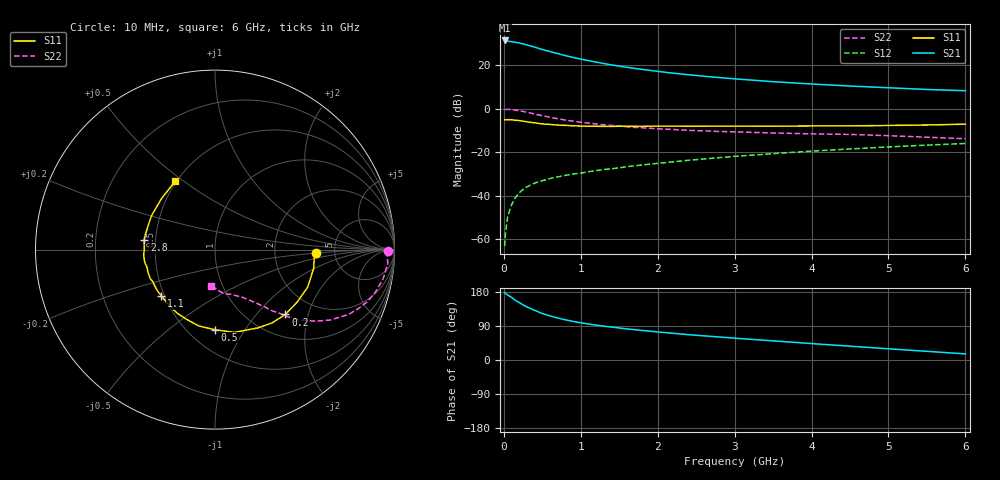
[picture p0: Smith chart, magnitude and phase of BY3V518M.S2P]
! SIEMENS Small Signal Semiconductors
! BFY420
! Si NPN RF SIEGET Grounded Emitter Transistor in MICRO-X
! VCE = 3.5 V  IC = 18 mA
! Common Emitter S-Parameters:  October  1996
# GHz  S  MA  R  50
!  f  S11  S21  S12  S22
! GHz  MAG  ANG  MAG  ANG  MAG  ANG  MAG  ANG
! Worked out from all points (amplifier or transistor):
!   36 points, 10 MHz to 6 GHz, reference 50 ohm
!   highest |S21| = 31.3 dB at 10 MHz (marker M1)
!   |S21| within 3 dB of that: start of sweep to 395.2 MHz
!   unconditionally stable (mu >= 1): start of sweep to 12.51 MHz; 2.07 GHz to end of sweep
!   at 250 MHz: K = 0.29, MSG = 33.4 dB, |S12| = -37.1 dB
!   at 1.4 GHz: K = 0.89, MSG = 23.8 dB, |S12| = -27.6 dB
!   at 6 GHz: K = 1.06, MAG = 10.6 dB, |S12| = -16.0 dB
!   S11 on the Smith chart (normalised r, x): 10 MHz: 3.55, -0.21; 200 MHz: 1.43, -1.45; 500 MHz: 0.67, -0.74; 1.1 GHz: 0.48, -0.29; 2.8 GHz: 0.43, +0.06; 6 GHz: 0.49, +0.46
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0.01  0.5616 -2.1  36.71 178.4  0.0007 72.9  0.9626 -0.5
0.02  0.5546 -4.5  36.18 175.7  0.0013 71.8  0.9589 -1.4
0.1  0.5572 -22.1  34.53 165.2  0.0062 80.8  0.951 -9.8
0.15  0.543 -32.6  33.32 157.4  0.0091 71.7  0.9268 -14.5
0.2  0.5334 -42.6  32.09 151.7  0.0118 72.0  0.8983 -18.7
0.25  0.5174 -52.2  30.55 145.3  0.014 69.2  0.8616 -22.6
0.3  0.4976 -61.2  28.98 139.9  0.0161 67.3  0.8267 -25.9
0.4  0.4736 -76.8  25.85 131.1  0.0196 63.4  0.7528 -31.4
0.5  0.4461 -90.2  22.76 122.6  0.0222 60.1  0.6883 -35.4
0.6  0.435 -101.9  20.4 116.4  0.0249 58.4  0.634 -38.5
0.7  0.4206 -111.2  18.36 110.8  0.0272 58.6  0.5882 -41.1
0.8  0.413 -119.9  16.49 106.0  0.0294 56.8  0.5479 -42.9
0.9  0.4056 -126.6  14.96 101.9  0.0317 56.9  0.5159 -44.1
1.1  0.395 -139.2  12.67 95.0  0.0357 57.0  0.4661 -47.0
1.3  0.3924 -148.3  10.84 89.3  0.0402 57.0  0.4275 -48.7
1.6  0.3943 -160.2  8.885 82.0  0.0466 57.4  0.3838 -51.7
2.2  0.3987 -175.9  6.518 70.5  0.0602 56.5  0.3329 -56.7
2.8  0.3982 172.1  5.172 60.7  0.0752 54.1  0.2989 -61.3
3.5  0.3959 159.7  4.159 50.5  0.0928 50.2  0.2767 -66.7
4.5  0.4026 144.4  3.301 36.5  0.1189 42.8  0.2561 -75.2
5.5  0.4223 127.9  2.754 22.9  0.1457 34.3  0.2214 -87.7
6  0.4405 120.4  2.58 16.1  0.1589 29.7  0.2041 -95.8
